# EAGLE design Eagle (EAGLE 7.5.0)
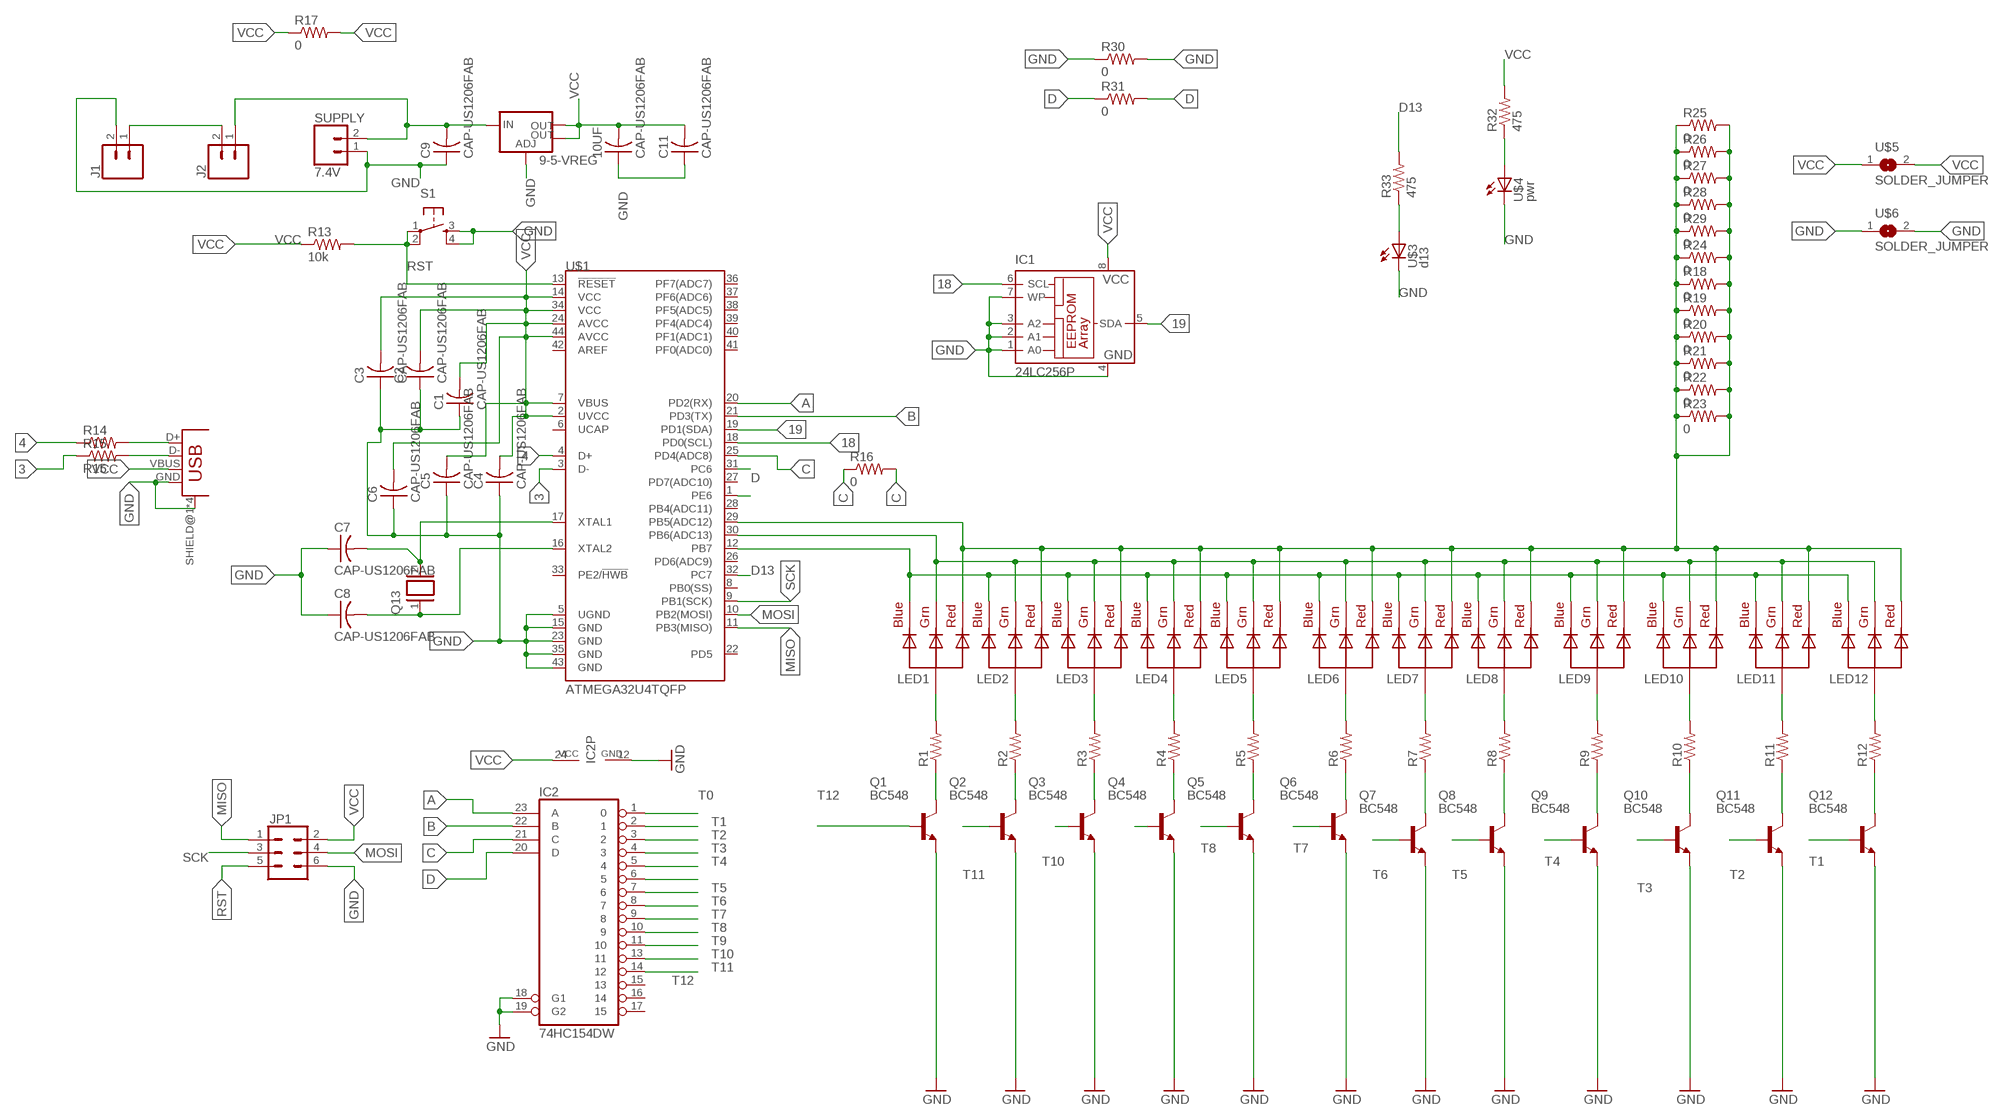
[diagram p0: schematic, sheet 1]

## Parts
9-5-VREG  V_REG_LM1117SOT223  [SOT223]
10UF  CAP-US1206FAB  [C1206FAB]
C1  CAP-US1206FAB  [C1206FAB]
C2  CAP-US1206FAB  [C1206FAB]
C3  CAP-US1206FAB  [C1206FAB]
C4  CAP-US1206FAB  [C1206FAB]
C5  CAP-US1206FAB  [C1206FAB]
C6  CAP-US1206FAB  [C1206FAB]
C7  CAP-US1206FAB  [C1206FAB]
C8  CAP-US1206FAB  [C1206FAB]
C9  CAP-US1206FAB  [C1206FAB]
C11  CAP-US1206FAB  [C1206FAB]
IC1  24LC256P  [DIL8]
IC2  74HC154DW  [SO24W]
J1  CONN_02  [1X02]
J2  CONN_02  [1X02]
JP1  CONN_03X22X3_SILK_MALE_PTH  [2X3]
LED1  RGBLED_CA-5MM  [LED5MMRGB]
LED2  RGBLED_CA-5MM  [LED5MMRGB]
LED3  RGBLED_CA-5MM  [LED5MMRGB]
LED4  RGBLED_CA-5MM  [LED5MMRGB]
LED5  RGBLED_CA-5MM  [LED5MMRGB]
LED6  RGBLED_CA-5MM  [LED5MMRGB]
LED7  RGBLED_CA-5MM  [LED5MMRGB]
LED8  RGBLED_CA-5MM  [LED5MMRGB]
LED9  RGBLED_CA-5MM  [LED5MMRGB]
LED10  RGBLED_CA-5MM  [LED5MMRGB]
LED11  RGBLED_CA-5MM  [LED5MMRGB]
LED12  RGBLED_CA-5MM  [LED5MMRGB]
Q1  BC548  [TO92-EBC]
Q2  BC548  [TO92-EBC]
Q3  BC548  [TO92-EBC]
Q4  BC548  [TO92-EBC]
Q5  BC548  [TO92-EBC]
Q6  BC548  [TO92-EBC]
Q7  BC548  [TO92-EBC]
Q8  BC548  [TO92-EBC]
Q9  BC548  [TO92-EBC]
Q10  BC548  [TO92-EBC]
Q11  BC548  [TO92-EBC]
Q12  BC548  [TO92-EBC]
Q13  XTAL  [Q]
R1  R-US_0207/10  [0207/10]
R2  R-US_0207/10  [0207/10]
R3  R-US_0207/10  [0207/10]
R4  R-US_0207/10  [0207/10]
R5  R-US_0207/10  [0207/10]
R6  R-US_0207/10  [0207/10]
R7  R-US_0207/10  [0207/10]
R8  R-US_0207/10  [0207/10]
R9  R-US_0207/10  [0207/10]
R10  R-US_0207/10  [0207/10]
R11  R-US_0207/10  [0207/10]
R12  R-US_0207/10  [0207/10]
R13  10k  RES-US1206FAB  [R1206FAB]
R14  RES-US1206FAB  [R1206FAB]
R15  R15  RES-US1206FAB  [R1206FAB]
R16  0  RES-US1206FAB  [R1206FAB]
R17  0  RES-US1206FAB  [R1206FAB]
R18  0  RES-US1206FAB  [R1206FAB]
R19  0  RES-US1206FAB  [R1206FAB]
R20  0  RES-US1206FAB  [R1206FAB]
R21  0  RES-US1206FAB  [R1206FAB]
R22  0  RES-US1206FAB  [R1206FAB]
R23  0  RES-US1206FAB  [R1206FAB]
R24  0  RES-US1206FAB  [R1206FAB]
R25  0  RES-US1206FAB  [R1206FAB]
R26  0  RES-US1206FAB  [R1206FAB]
R27  0  RES-US1206FAB  [R1206FAB]
R28  0  RES-US1206FAB  [R1206FAB]
R29  0  RES-US1206FAB  [R1206FAB]
R30  0  RES-US1206FAB  [R1206FAB]
R31  0  RES-US1206FAB  [R1206FAB]
R32  475  RES-US1206FAB  [R1206FAB]
R33  475  RES-US1206FAB  [R1206FAB]
S1  6MM_SWITCH6MM_SWITCH  [6MM_SWITCH]
SUPPLY  7.4V  CONN_02  [1X02]
U$1  ATMEGA32U4TQFP  [SPARKFUN-DIGITALIC_TQFP44]
U$2  USB_MINIB  [USB_MINIB]
U$3  d13  LEDFAB1206  [LED1206FAB]
U$4  pwr  LEDFAB1206  [LED1206FAB]
U$5  SOLDER_JUMPER  [SJFAB]
U$6  SOLDER_JUMPER  [SJFAB]

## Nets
3: R15.1 U$1.3(D-)
4: R14.1 U$1.4(D+)
18: IC1.6(SCL) U$1.18(PD0(SCL))
19: IC1.5(SDA) U$1.19(PD1(SDA))
A: IC2.23(A) U$1.20(PD2(RX))
B: IC2.22(B) U$1.21(PD3(TX))
C: IC2.21(C) R16.1 R16.2 U$1.25(PD4(ADC8))
D: IC2.20(D) R31.1 R31.2 U$1.1(PE6)
D13: R33.2 U$1.32(PC7)
GND: 9-5-VREG.1(ADJ) 10UF.1 C1.1 C2.1 C3.1 C4.1 C5.1 C6.1 C7.1 C8.1 C9.1 C11.1 IC1.1(A0) IC1.2(A1) IC1.3(A2) IC1.4(GND) IC1.7(WP) IC2.12(GND) IC2.18(G1) IC2.19(G2) J1.2 JP1.6 Q1.E Q2.E Q3.E Q4.E Q5.E Q6.E Q7.E Q8.E Q9.E Q10.E Q11.E Q12.E R30.1 R30.2 S1.3(S) S1.4(S1) SUPPLY.1 U$1.5(UGND) U$1.15(GND) U$1.23(GND) U$1.35(GND) U$1.43(GND) U$2.GND U$2.SHIELD@1(SHIELD) U$2.SHIELD@2(SHIELD) U$2.SHIELD@3(SHIELD) U$2.SHIELD@4(SHIELD) U$3.2(C) U$4.2(C) U$6.1 U$6.2
MISO: JP1.1 U$1.11(PB3(MISO))
MOSI: JP1.4 U$1.10(PB2(MOSI))
N$1: J1.1 J2.2
N$2: R32.1 U$4.1(A)
N$3: U$1.31(PC6)
N$4: 9-5-VREG.3(IN) C9.2 J2.1 SUPPLY.2
N$5: R33.1 U$3.1(A)
N$6: LED1.1(RED) LED2.1(RED) LED3.1(RED) LED4.1(RED) LED5.1(RED) LED6.1(RED) LED7.1(RED) LED8.1(RED) LED9.1(RED) LED10.1(RED) LED11.1(RED) LED12.1(RED) R18.1 R18.2 R19.1 R19.2 R20.1 R20.2 R21.1 R21.2 R22.1 R22.2 R23.1 R23.2 R24.1 R24.2 R25.1 R25.2 R26.1 R26.2 R27.1 R27.2 R28.1 R28.2 R29.1 R29.2 U$1.29(PB5(ADC12))
N$12: C7.2 Q13.2 U$1.17(XTAL1)
N$13: C8.2 Q13.1 U$1.16(XTAL2)
N$14: R14.2 U$2.D+
N$15: R15.2 U$2.D-
N$16: Q1.C R1.1
N$17: Q2.C R2.1
N$18: Q3.C R3.1
N$19: Q4.C R4.1
N$20: Q5.C R5.1
N$21: Q6.C R6.1
N$22: Q7.C R7.1
N$23: Q8.C R8.1
N$24: Q9.C R9.1
N$25: Q10.C R10.1
N$26: Q11.C R11.1
N$27: Q12.C R12.1
N$29: LED1.3(GREEN) LED2.3(GREEN) LED3.3(GREEN) LED4.3(GREEN) LED5.3(GREEN) LED6.3(GREEN) LED7.3(GREEN) LED8.3(GREEN) LED9.3(GREEN) LED10.3(GREEN) LED11.3(GREEN) LED12.3(GREEN) U$1.30(PB6(ADC13))
N$31: LED1.2(VCC) R1.2
N$32: LED2.2(VCC) R2.2
N$33: LED3.2(VCC) R3.2
N$34: LED4.2(VCC) R4.2
N$35: LED5.2(VCC) R5.2
N$36: LED6.2(VCC) R6.2
N$37: LED7.2(VCC) R7.2
N$38: LED8.2(VCC) R8.2
N$39: LED9.2(VCC) R9.2
N$40: LED10.2(VCC) R10.2
N$41: LED11.2(VCC) R11.2
N$42: LED12.2(VCC) R12.2
N$46: LED1.4(BLUE) LED2.4(BLUE) LED3.4(BLUE) LED4.4(BLUE) LED5.4(BLUE) LED6.4(BLUE) LED7.4(BLUE) LED8.4(BLUE) LED9.4(BLUE) LED10.4(BLUE) LED11.4(BLUE) LED12.4(BLUE) U$1.12(PB7)
RST: JP1.5 R13.2 S1.1(P) S1.2(P1) U$1.13(!RESET)
SCK: JP1.3 U$1.9(PB1(SCK))
T0: IC2.1
T1: IC2.2 Q12.B
T2: IC2.3 Q11.B
T3: IC2.4 Q10.B
T4: IC2.5 Q9.B
T5: IC2.6 Q8.B
T6: IC2.7 Q7.B
T7: IC2.8 Q6.B
T8: IC2.9 Q5.B
T9: IC2.10 Q4.B
T10: IC2.11 Q3.B
T11: IC2.13 Q2.B
T12: IC2.14 Q1.B
VCC: 9-5-VREG.2(OUT) 9-5-VREG.4(OUT) 10UF.2 C1.2 C2.2 C3.2 C4.2 C5.2 C6.2 C11.2 IC1.8(VCC) IC2.24(VCC) JP1.2 R13.1 R17.1 R17.2 R32.2 U$1.2(UVCC) U$1.7(VBUS) U$1.14(VCC) U$1.24(AVCC) U$1.34(VCC) U$1.44(AVCC) U$2.VBUS U$5.1 U$5.2
Unconnected: IC2.15 IC2.16 IC2.17 U$1.6(UCAP) U$1.8(PB0(SS)) U$1.22(PD5) U$1.26(PD6(ADC9)) U$1.27(PD7(ADC10)) U$1.28(PB4(ADC11)) U$1.33(PE2/!HWB) U$1.36(PF7(ADC7)) U$1.37(PF6(ADC6)) U$1.38(PF5(ADC5)) U$1.39(PF4(ADC4)) U$1.40(PF1(ADC1)) U$1.41(PF0(ADC0)) U$1.42(AREF)

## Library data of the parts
9-5-VREG = fab:V_REG_LM1117: Voltage Regulator LM1117 Standard adjustable voltage regulator but in SMD form. Spark Fun Electronics SKU : COM-00595; PROD_ID: VREG-08170
10UF C1-C9 C11 = fab:CAP-US
IC1 = microchip:24*: Serial EEPROM I2C; MF: MICROCHIP; MPN: 24LC256-E/P; OC_FARNELL: 9757970; OC_NEWARK: 92C7169
IC2 = 74xx-eu:74*154: 4-line to 16-line data SELECTOR/MULTIPLEXER
J1 J2 SUPPLY = SparkFun-Connectors:CONN_02: Multi connection point. Often used as Generic Header-pin footprint for 0.1 inch spaced/style header connections
JP1 = SparkFun-Connectors:CONN_03X2: Multi connection point. Often used as Generic Header-pin footprint for 0.1 inch spaced/style header connections You can populate with any combo of single row headers, but if you'd like an exact match, check these: Header - 2x3 (Male, 0.1") (PRT-12807) Header - 2x3 (Female, 0.1") (PRT-13010) 2x3 Pin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; PROD_ID: CONN-09701
LED1-LED12 = adafruitModified:RGBLED_CA: RGB LED, common-anode 5MM Staggered pins 5mm Piranha package http://www.ladyada.net/library/pcb/eaglelibrary.html
Q1-Q12 = transistor-npn:BC548*: NPN Transistor
Q13 = special:XTAL: CRYSTAL
R1-R12 = adafruit:R-US_: RESISTOR, American symbol
R13-R33 = fab:RES-US: Resistor (US Symbol)
S1 = fab:6MM_SWITCH: OMRON SWITCH
U$1 = SparkFun-Retired:ATMEGA32U4: Atmel 44-pin 8-bit Microcontroller with 32KBytes of ISP Flash and USB Controller ----- Please use the QFN-44-NOPAD_1:1 package for the footprint of all boards using a 32U4. Route traces directly away from the pads as much as possible.; PROD_ID: IC-11161
U$2 = fab:USB_MINIB
U$3 U$4 = fab:LED: LED
U$5 U$6 = fab:SOLDER_JUMPER

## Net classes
0 default: drill 0.406 mm, clearance 0.305 mm

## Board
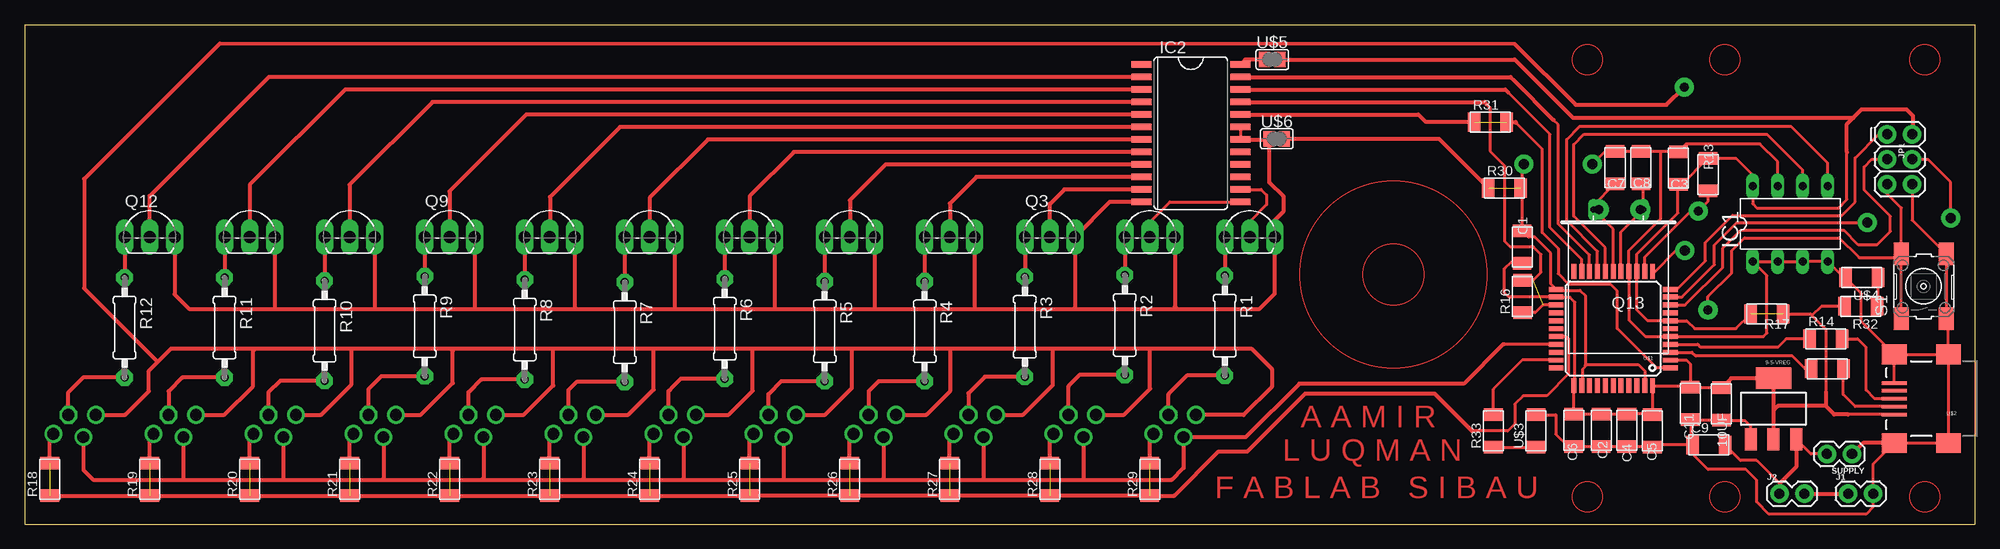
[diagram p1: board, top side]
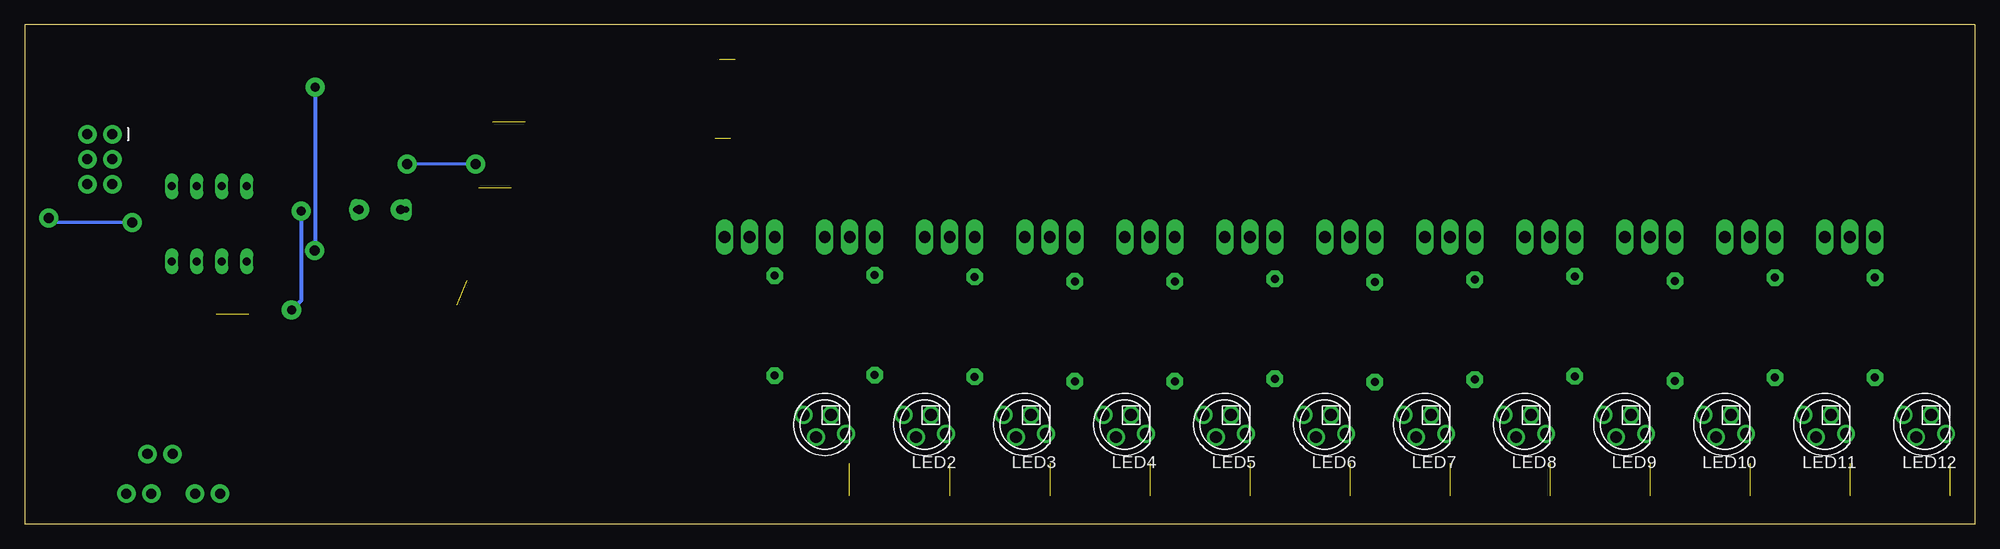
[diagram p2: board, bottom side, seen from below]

Size 198.12 x 50.8 mm. Coordinates in mm from the lower left corner, seen from the top.
Outline: 0,50.8 198.12,50.8 198.12,0 0,0 0,50.8
Copper layers (1*16): Top 0.035mm / dielectric 1.5mm / Bottom 0.035mm
Design rules "default *": minimum track width 10mil, minimum drill 24mil, track to track 12mil, track to pad 12mil, pad to pad 12mil, via to via 12mil, smd to smd 12mil, copper to edge 40mil, drill to drill 8mil, minimum pad ring 10mil, minimum via ring 8mil, stop-mask expansion 4mil, vias tented up to drill 0mil, thermal gap 10mil

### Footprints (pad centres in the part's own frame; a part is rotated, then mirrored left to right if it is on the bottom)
SOT223 = smd 1.219 x 2.235: 1 -2.311,-3.099; 2 0,-3.099; 3 2.311,-3.099 | smd 3.6 x 2.2: 4 0,3.099
C1206FAB = smd 1.27 x 1.905: 1 -1.651,0; 2 1.651,0
DIL8 = drill 0.813 long: 1 -3.81,-3.81; 2 -1.27,-3.81; 3 1.27,-3.81; 4 3.81,-3.81; 5 3.81,3.81; 6 1.27,3.81; 7 -1.27,3.81; 8 -3.81,3.81
SO24W = smd 0.66 x 2.032: 1 -6.985,-5.029; 2 -5.715,-5.029; 3 -4.445,-5.029; 4 -3.175,-5.029; 5 -1.905,-5.029; 6 -0.635,-5.029; 7 0.635,-5.029; 8 1.905,-5.029; 9 3.175,-5.029; 10 4.445,-5.029; 11 5.715,-5.029; 12 6.985,-5.029; 13 6.985,5.029; 14 5.715,5.029; 15 4.445,5.029; 16 3.175,5.029; 17 1.905,5.029; 18 0.635,5.029; 19 -0.635,5.029; 20 -1.905,5.029; 21 -3.175,5.029; 22 -4.445,5.029; 23 -5.715,5.029; 24 -6.985,5.029
1X02 = drill 1.016 pad 1.88: 1 0,0; 2 2.54,0
2X3 = drill 1.016 pad 1.88: 1 0,0; 2 0,2.54; 3 2.54,0; 4 2.54,2.54; 5 5.08,0; 6 5.08,2.54
LED5MMRGB = drill 1.2 pad 1.778: 1 -2.159,0.968; 3 0.889,1.286; 4 2.159,-0.968 | drill 1.2 pad 1.778 octagon: 2 -0.635,-0.968
TO92-EBC = drill 1.2 long: B 0,-1.27; C -2.54,-1.27; E 2.54,-1.27
Q = drill 0.61 long: 1 -2.54,-7.62; 2 2.54,-7.62
0207/10 = drill 0.813 pad 1.676 octagon: 1 -5.08,0; 2 5.08,0
R1206FAB = smd 1.27 x 1.905: 1 -1.651,0; 2 1.651,0
6MM_SWITCH = smd 2.286 x 1.524: 1 -3.302,2.286; 2 3.302,2.286; 3 -3.302,-2.286; 4 3.302,-2.286
SPARKFUN-DIGITALIC_TQFP44 = smd 1.5 x 0.5: 1 -5.8,4; 2 -5.8,3.2; 3 -5.8,2.4; 4 -5.8,1.6; 5 -5.8,0.8; 6 -5.8,0; 7 -5.8,-0.8; 8 -5.8,-1.6; 9 -5.8,-2.4; 10 -5.8,-3.2; 11 -5.8,-4; 23 5.8,-4; 24 5.8,-3.2; 25 5.8,-2.4; 26 5.8,-1.6; 27 5.8,-0.8; 28 5.8,0; 29 5.8,0.8; 30 5.8,1.6; 31 5.8,2.4; 32 5.8,3.2; 33 5.8,4 | smd 0.5 x 1.5: 12 -4,-5.8; 13 -3.2,-5.8; 14 -2.4,-5.8; 15 -1.6,-5.8; 16 -0.8,-5.8; 17 0,-5.8; 18 0.8,-5.8; 19 1.6,-5.8; 20 2.4,-5.8; 21 3.2,-5.8; 22 4,-5.8; 34 4,5.8; 35 3.2,5.8; 36 2.4,5.8; 37 1.6,5.8; 38 0.8,5.8; 39 0,5.8; 40 -0.8,5.8; 41 -1.6,5.8; 42 -2.4,5.8; 43 -3.2,5.8; 44 -4,5.8
USB_MINIB = smd 2.5 x 0.35: D+ 3.77,0; D- 3.77,0.8; GND 3.77,-1.6; ID 3.77,-0.8; VBUS 3.77,1.6 | smd 2.5 x 2: SHIELD@1 -1.73,-4.5; SHIELD@2 -1.73,4.5; SHIELD@3 3.77,4.5; SHIELD@4 3.77,-4.5
LED1206FAB = smd 1.27 x 1.905: 1 -1.651,0; 2 1.651,0
SJFAB = smd 1.118 x 1.6: 1 -0.787,0; 2 0.787,0

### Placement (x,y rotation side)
9-5-VREG  177.65,11.76 0 top
10UF  172.38,12.22 90 top
C1  152.13,28.21 270 top
C2  160.16,9.55 90 top
C3  168.01,36.2 270 top
C4  162.76,9.55 90 top
C5  165.36,9.49 90 top
C6  157.37,9.55 90 top
C7  161.57,36.27 270 top
C8  164.2,36.27 270 top
C9  171.08,8.06 0 top
C11  169.19,12.29 90 top
IC1  179.35,30.55 0 top
IC2  118.47,39.76 270 top
J1  185.25,3.12 0 top
J2  178.27,3.12 0 top
JP1  189.22,39.65 270 top
LED1  116.84,10.16 180 bottom
LED2  106.68,10.16 180 bottom
LED3  96.52,10.16 180 bottom
LED4  86.36,10.16 180 bottom
LED5  76.2,10.16 180 bottom
LED6  66.04,10.16 180 bottom
LED7  55.88,10.16 180 bottom
LED8  45.72,10.16 180 bottom
LED9  35.56,10.16 180 bottom
LED10  25.4,10.16 180 bottom
LED11  15.24,10.16 180 bottom
LED12  5.08,10.16 180 bottom
Q1  124.46,30.48 0 top
Q2  114.3,30.48 0 top
Q3  104.14,30.48 0 top
Q4  93.98,30.48 0 top
Q5  83.82,30.48 0 top
Q6  73.66,30.48 0 top
Q7  63.5,30.48 0 top
Q8  53.34,30.48 0 top
Q9  43.18,30.48 0 top
Q10  33.02,30.48 0 top
Q11  22.86,30.48 0 top
Q12  12.7,30.48 0 top
Q13  161.92,24.38 180 top
R1  121.92,20.2 270 top
R2  111.76,20.26 270 top
R3  101.6,20.07 270 top
R4  91.44,19.61 270 top
R5  81.28,19.61 270 top
R6  71.12,19.87 270 top
R7  60.96,19.55 270 top
R8  50.8,19.81 270 top
R9  40.64,20.13 270 top
R10  30.48,19.68 270 top
R11  20.32,20 270 top
R12  10.16,20 270 top
R13  171.01,35.55 270 top
R14  182.97,18.87 0 top
R15  183.1,15.82 0 top
R16  152.16,23.14 90 top
R17  177,21.39 180 top
R18  2.54,4.57 90 top
R19  12.7,4.57 90 top
R20  22.86,4.57 90 top
R21  33.02,4.57 90 top
R22  43.18,4.57 90 top
R23  53.34,4.57 90 top
R24  63.5,4.57 90 top
R25  73.66,4.57 90 top
R26  83.82,4.57 90 top
R27  93.98,4.57 90 top
R28  104.14,4.57 90 top
R29  114.3,4.57 90 top
R30  150.34,34.19 0 top
R31  148.91,40.88 0 top
R32  186.55,22.16 180 top
R33  149.22,9.49 90 top
S1  192.91,24.18 90 top
SUPPLY  185.64,7.15 180 top
U$1  161.38,19.89 180 top
U$2  193.7,12.77 180 top
U$3  153.53,9.49 90 top
U$4  186.62,25.09 180 top
U$5  126.75,47.26 0 top
U$6  127.2,39.2 0 top

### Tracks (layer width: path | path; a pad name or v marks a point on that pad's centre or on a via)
3
  Top 0.305: U$1.3 169.38,17.49 169.78,17.09 179.59,17.09 180.96,15.73 181.37,15.73 R15.1
4
  Top 0.305: U$1.4 169.95,18.29 170.24,18 178.1,18 178.96,18.87 R14.1
18
  Top 0.305: U$1.18 160.57,28.12 157.37,31.33 157.37,38.61 158.41,39.65 177,39.65 180.62,36.02 IC1.6
19
  Top 0.305: U$1.19 159.78,27.75 156.65,30.88 156.65,39.13 157.95,40.43 179.47,40.43 183.16,36.73 IC1.5
A
  Top 0.305: U$1.20 158.97,27.38 155.81,30.55 155.81,40.62 155.32,41.11 | 151.29,45.14 151.06,45.37
  Top 0.406: 155.32,41.11 151.29,45.14 150.96,45.48 IC2.23
B
  Top 0.305: U$1.21 158.18,26.95 154.96,30.16 154.96,39.65 150.7,43.91 150.47,44.13 149.24,44.13
  Top 0.406: IC2.22 150.41,44.2 150.7,43.91
C  (1 unrouted)
  Top 0.305: U$1.25 154.24,22.29 153.47,21.52 152.19,21.52 R16.1 | R16.2 153.23,24.79 154.05,25.61 154.05,27.43 153.27,28.21 150.93,28.21 150.34,28.8 150.34,36.47 148.85,37.96 148.85,42.38 148.53,42.7 148.36,42.87
  Top 0.406: IC2.21 148.29,42.94 148.53,42.7
D  (1 unrouted)
  Top 0.305: 151.51,40.82 154.18,38.16 154.18,29.64 155.81,28.02 155.81,25.48 156.84,24.44 161.07,24.44 161.78,23.73 161.78,19.89 165.78,15.89 U$1.1
  Top 0.406: IC2.20 141.57,41.66 142.35,40.88 R31.1 | R31.2 151.45,40.88 151.51,40.82
D13
  Top 0.305: U$1.32 152.15,16.69 149.22,13.76 R33.2
GND  (via drill 1.02 pad 1.93)  (3 unrouted)
  Top 0.305: C5.1 165.29,7.9 C4.1 C2.1 C6.1 156.81,7.9 155.54,9.16 155.54,11.12 155.52,11.14 U$3.2 | U$2.GND U$2.SHIELD@4 | IC2.19 IC2.18 | IC1.1 IC1.2 IC1.3 IC1.4 184.81,25.09 U$4.2 186.6,23.46 186.6,20.61 U$2.SHIELD@4 | U$2.SHIELD@1 U$2.SHIELD@2 U$2.SHIELD@3 187.79,6.14 J1.2 187.79,1.76 187.07,1.04 177.19,1.04 175.96,2.27 175.96,4.49 174.85,5.59 171.01,5.59 169.59,7.02 169.59,7.9 C9.1 | 165.4,7.8 C5.1 | U$2.SHIELD@4 189.92,16.59 | 166.21,37.92 C8.1 C7.1 160.58,37.92 v159.25,36.59 | 166.21,37.92 167.9,37.92 C3.1 168.78,38.67 176.28,38.67 178.09,36.87 IC1.7 | IC2.12 | 152.13,33.97 C1.1 152.8,29.18 153.4,29.18 155.03,27.56 155.03,24.44 155.56,23.9 | 152.13,33.97 151.91,34.19 | 152.13,33.97 152.13,36.43 v152.29,36.59 | U$2.SHIELD@4 U$2.SHIELD@1 | 194.88,17.14 U$2.SHIELD@1 | S1.4 S1.3 195.43,20.64 U$2.SHIELD@1 | S1.4 194.88,28.07 | 175.89,26.39 IC1.1 | 189.87,17.16 189.87,16.66 U$2.SHIELD@4 | 169.26,10.57 10UF.1 172.42,10.53 174.78,10.53 175.33,9.98 9-5-VREG.1 | 169.26,10.57 C11.1 | IC1.1 177,25.29 177,19.43 176.65,19.09 U$1.5 164.66,19.09 162.97,20.78 U$1.15 162.97,27.84 166.21,31.07 166.21,37.92 | 169.26,10.57 169.26,8.23 C9.1 | C9.1 165.58,8.06 C5.1 | JP1.6 191.75,30.92 S1.4 | U$1.43 164.58,15.6 163.93,16.25 158.6,16.25 158.53,16.18 | 155.5,23.9 155.56,23.9 | 155.56,23.9 U$1.23 | 155.56,23.9 156.08,23.9 156.19,23.79 158.01,23.79 158.53,23.27 158.53,16.18 | 158.53,16.18 158.53,16.05 158.28,15.79 158.28,14.76 158.18,14.65 U$1.35
  Top 0.406: U$2.SHIELD@3 186.76,8.27 SUPPLY.1 | Q12.E 15.24,23.37 16.7,21.91 25.48,21.91 | 25.48,21.91 35.62,21.91 | 35.62,21.91 45.76,21.91 | 45.76,21.91 56.03,21.91 | 56.03,21.91 66.17,21.91 | 66.17,21.91 76.18,21.91 | 76.18,21.91 86.39,21.91 | 86.39,21.91 96.59,21.91 | 96.59,21.91 106.8,21.91 | 106.8,21.91 117.06,21.91 | 117.06,21.91 125.45,21.91 127.01,23.46 Q1.E 127,30.93 127.86,31.79 127.86,33.34 126.42,34.78 U$6.1 126.35,39.12 IC2.18 | Q2.E 116.84,22.13 117.06,21.91 | 106.8,21.91 106.68,22.02 Q3.E 110.23,32.76 IC2.12 | Q4.E 96.52,21.98 96.59,21.91 | Q5.E 86.36,21.93 86.39,21.91 | Q6.E 76.2,21.93 76.18,21.91 | Q7.E 66.04,22.04 66.17,21.91 | Q8.E 55.88,22.05 56.03,21.91 | Q9.E 45.72,21.95 45.76,21.91 | Q10.E 35.56,21.96 35.62,21.91 | Q11.E 25.4,21.98 25.48,21.91 | U$6.2 143.69,39.2 R30.1
  Bottom 0.305: v152.29,36.59 v159.25,36.59
MISO
  Top 0.305: JP1.1 188.37,39.65 185.97,37.24 185.97,32.76 184.6,31.39 173.49,31.39 170.75,28.66 170.75,26.78 167.87,23.89 U$1.11
MOSI  (via drill 1.02 pad 1.93)
  Top 0.305: v195.65,31.14 195.65,34.77 193.31,37.11 JP1.4 | U$1.10 168.37,23.09 171.66,26.39 171.66,28.41 173.94,30.68 v187.2,30.68
  Bottom 0.305: v187.2,30.68 195.19,30.68 v195.65,31.14
N$1
  Top 0.406: J2.2 J1.1
N$2
  Top 0.305: U$4.1 188.27,22.23 R32.1
N$4
  Top 0.305: 178.29,4.16 175.96,6.5 174.29,6.5 C9.2 | SUPPLY.2 181.46,7.15 9-5-VREG.3
  Top 0.406: 9-5-VREG.3 179.96,5.82 178.29,4.16 178.29,3.14 J2.1
N$5
  Top 0.305: R33.1 U$3.1
N$6  (12 unrouted)
  Top 0.305: U$1.29 156.6,19.09 156.84,18.85 156.84,15.28 154.63,13.06 152.23,13.06 151.38,12.22 151.38,10.21 150.67,9.49 147.03,9.49
  Top 0.406: R18.2 2.54,8.81 LED12.1 | R19.2 12.7,8.81 LED11.1 | R20.2 22.86,8.81 LED10.1 | R21.2 33.02,8.81 LED9.1 | R22.2 43.18,8.81 LED8.1 | R23.2 53.34,8.81 LED7.1 | R24.2 63.5,8.81 LED6.1 | R25.2 73.66,8.81 LED5.1 | R26.2 83.82,8.81 LED4.1 | R27.2 93.98,8.81 LED3.1 | R28.2 104.14,8.81 LED2.1 | R29.2 114.3,8.81 LED1.1 | R18.1 R19.1 R20.1 R21.1 R22.1 R23.1 R24.1 R25.1 R26.1 R27.1 R28.1 R29.1 116.8,2.92 121.29,7.41 124.22,7.41 130.06,13.26 143.26,13.26 147.03,9.49
N$7  (via drill 0.91 pad 2.03)
  other vias: 164.12,31.98
N$8  (via drill 0.91 pad 2.03)
  other vias: 159.9,31.98
N$12
  Top 0.305: U$1.17 161.38,30 Q13.2 159.38,32.43 C7.2
N$13
  Top 0.305: U$1.16 162.18,29.71 Q13.1 164.46,34.37 C8.2
N$14
  Top 0.305: U$2.D+ 187.95,12.77 187.07,13.65 187.07,18 186.21,18.87 R14.2
N$15
  Top 0.305: 184.66,15.05 R15.2 184.73,15.12 184.73,13.2 185.95,11.97 U$2.D-
N$16
  Top 0.406: Q1.C R1.1
N$17
  Top 0.406: Q2.C R2.1
N$18
  Top 0.406: Q3.C R3.1
N$19
  Top 0.406: Q4.C R4.1
N$20
  Top 0.406: Q5.C R5.1
N$21
  Top 0.406: Q6.C R6.1
N$22
  Top 0.406: Q7.C R7.1
N$23
  Top 0.406: Q8.C R8.1
N$24
  Top 0.406: Q9.C R9.1
N$25
  Top 0.406: Q10.C R10.1
N$26
  Top 0.406: Q11.C R11.1
N$27
  Top 0.406: Q12.C R12.1
N$29
  Top 0.305: U$1.30 150.31,18.29
  Top 0.406: LED12.3 5.97,5.54 6.96,4.55 16.12,4.55 | 16.12,4.55 26.26,4.55 | 26.26,4.55 36.53,4.55 | 36.53,4.55 46.48,4.55 | 46.48,4.55 56.88,4.55 | 56.88,4.55 66.82,4.55 | 66.82,4.55 77.03,4.55 | 77.03,4.55 87.36,4.55 | 87.36,4.55 97.37,4.55 | 97.37,4.55 107.64,4.55 | 107.64,4.55 116.55,4.55 117.73,5.73 LED1.3 124.05,8.87 129.48,14.3 146.19,14.3 150.18,18.29 150.31,18.29 | LED11.3 16.13,4.56 16.12,4.55 | LED10.3 26.29,4.58 26.26,4.55 | LED9.3 36.45,4.63 36.53,4.55 | LED8.3 46.61,4.68 46.48,4.55 | LED7.3 56.77,4.66 56.88,4.55 | LED6.3 66.93,4.66 66.82,4.55 | LED5.3 77.09,4.61 77.03,4.55 | LED4.3 87.25,4.66 87.36,4.55 | LED3.3 97.41,4.59 97.37,4.55 | LED2.3 107.57,4.62 107.64,4.55
N$31
  Top 0.406: R1.2 118.08,15.12 116.2,13.24 LED1.2
N$32
  Top 0.406: R2.2 107.16,15.18 106.05,14.07 LED2.2
N$33
  Top 0.406: R3.2 97.54,14.99 95.88,13.32 LED3.2
N$34
  Top 0.406: R4.2 86.75,14.53 85.73,13.52 85.73,11.14 LED4.2
N$35
  Top 0.406: R5.2 76.87,14.53 75.56,13.23 LED5.2
N$36
  Top 0.406: R6.2 66.66,14.79 65.84,13.97 65.45,13.59 65.41,13.54 LED6.2
N$37
  Top 0.406: R7.2 56.07,14.47 55.24,13.64 LED7.2
N$38
  Top 0.406: R8.2 46.38,14.73 45.09,13.43 LED8.2
N$39
  Top 0.406: R9.2 36.24,15.05 34.91,13.71 34.91,11.15 LED9.2
N$40
  Top 0.406: R10.2 25.97,14.6 24.77,13.39 LED10.2
N$41
  Top 0.406: R11.2 16.03,14.92 14.62,13.52 14.62,11.15 LED11.2
N$42
  Top 0.406: R12.2 5.95,14.92 4.45,13.41 LED12.2
N$46  (via drill 0.91 pad 1.93, 1.02 pad 1.93)
  Top 0.305: U$1.12 165.29,25.61 165.56,25.61 167.76,27.82 v168.68,27.82
  Top 0.406: v168.61,44.46 166.79,42.64 157.56,42.64 151.38,48.81 19.82,48.88 6.04,35.1 6.04,23.98 13.52,16.51 | LED12.4 10.22,11.13 12.61,13.52 12.61,15.6 13.52,16.51 | 13.52,16.51 14.88,17.88 23.46,17.88 | 23.46,17.88 33.22,17.88 | 33.22,17.88 43.23,17.88 | 43.23,17.88 53.69,17.88 | 53.69,17.88 63.96,17.88 | 63.96,17.88 73.91,17.88 | 73.91,17.88 83.85,17.88 | 83.85,17.88 94.06,17.88 | 94.06,17.88 104.33,17.88 | 104.33,17.88 114.47,17.88 | 114.47,17.88 124.61,17.88 126.69,15.79 126.69,13.97 123.83,11.12 119.01,11.12 LED1.4 | LED11.4 20.29,11.13 23.2,14.04 23.2,17.61 23.46,17.88 | LED10.4 30.11,11.13 33.22,14.23 33.22,17.88 | LED9.4 40.25,11.13 43.48,14.37 43.48,17.61 43.23,17.88 | LED8.4 50.71,11.13 53.69,14.11 53.69,17.88 | LED7.4 61.31,11.13 63.9,13.71 63.9,17.81 63.96,17.88 | LED6.4 71.51,11.13 73.97,13.59 73.97,17.81 73.91,17.88 | LED5.4 81.33,11.13 84.05,13.85 84.05,17.68 83.85,17.88 | LED4.4 91.6,11.13 94.06,13.59 94.06,17.88 | LED3.4 101.41,11.13 104.45,14.17 104.45,17.75 104.33,17.88 | LED2.4 111.68,11.13 114.33,13.78 114.33,17.75 114.47,17.88
  Bottom 0.406: v168.61,44.46 168.61,27.89 v168.68,27.82
RST  (via drill 0.91 pad 1.93)
  Top 0.305: S1.1 S1.2 | S1.2 189.93,27.11 186.35,27.11 184.34,29.12 174.72,29.12 173.42,27.82 173.42,25.55 171.01,23.14 v171.01,21.77 | U$1.13 164.57,27.16 169.26,31.85 | R13.2 171.01,32.83 v170.04,31.85 | S1.2 190.63,27.48 190.65,27.5 190.65,32.17 189.09,33.73 189.09,34.44 JP1.5
  Top 0.406: 169.26,31.85 v170.04,31.85
  Bottom 0.406: v170.04,31.85 170.04,22.75 v171.01,21.77
SCK
  Top 0.305: U$1.9 168.67,22.29 172.51,26.13 172.51,28.08 174.33,29.9 184.79,29.9 186.29,28.41 188.18,28.41 189.54,29.77 189.54,31.33 186.88,33.99 186.88,36.34 187.66,37.12 JP1.3
T1
  Top 0.406: IC2.2 24.8,45.48 12.7,33.37 Q12.B
T2
  Top 0.406: IC2.3 32.57,44.2 22.88,34.52 22.88,29.23 Q11.B
T3
  Top 0.406: IC2.4 41.44,42.94 33.02,34.52 Q10.B
T4
  Top 0.406: IC2.5 50.96,41.66 43.16,33.87 43.16,29.23 Q9.B
T5
  Top 0.406: IC2.6 60.48,40.4 53.37,33.28 53.37,29.23 Q8.B
T6
  Top 0.406: IC2.7 69.42,39.12 63.51,33.22 Q7.B
T7
  Top 0.406: IC2.8 78.16,37.85 73.64,33.34 73.64,29.23 Q6.B
T8
  Top 0.406: IC2.9 87.48,36.59 83.85,32.95 83.85,29.24 Q5.B
T9
  Top 0.406: IC2.10 96.67,35.31 93.99,32.63 Q4.B
T10
  Top 0.406: IC2.11 105.62,34.05 104.14,32.56 Q3.B
T11
  Top 0.305: Q2.B 114.3,30.71 116.35,32.76 123.48,32.76 IC2.13
T12
  Top 0.305: Q1.B 124.46,30.8 126.17,32.5 126.17,33.48 125.59,34.05 IC2.14
VCC  (2 unrouted)
  Top 0.305: 157.37,13.59 C6.2 C2.2 C4.2 165.29,11.21 C5.2 165.38,11.16 U$1.44 169.04,14.09 C11.2 | 157.37,13.59 157.37,14.08 U$1.34 | 167.16,16.7 U$1.2 168.82,16.69 169.19,16.32 C11.2 | U$1.24 150.78,23.09 150.34,23.53 150.34,26 151.06,26.71 151.97,26.71 C1.2 | U$1.24 150.94,23.09 | 182.97,13.46 182.97,19.82 181.58,21.22 | 185.12,37.83 185.12,33.02 184.28,32.17 175.96,32.17 175.54,32.59 IC1.8 175.56,34.38 175.56,35.49 173.85,37.21 R13.1 168.3,34.49 168.03,34.49 C3.2 167.96,34.5 167.96,31.66 163.78,27.47 U$1.14 163.78,21.8 164.88,20.69 U$1.7 168.85,20.69 169.65,19.89 173.85,19.89 R17.2 | U$2.VBUS 185.26,11.17 | C11.2 172.31,13.94 10UF.2 | R17.1 181.41,21.39 181.58,21.22 | R32.2 182.52,22.16 181.58,21.22 | U$1.24 155.59,23.07 156.97,23.07 157.5,22.55 157.5,14.76 157.38,14.63 157.38,13.6 157.37,13.59
  Top 0.406: 185.77,41.34 157.3,41.34 151.38,47.26 U$5.2 | 185.77,41.34 186.62,42.19 191.16,42.19 191.81,41.53 191.81,39.71 JP1.2 | 185.12,37.83 185.12,40.69 185.77,41.34 | 10UF.2 173.36,14.85 9-5-VREG.4 177.71,14.79 177.71,11.63 | 177.71,11.63 177.71,8.72 9-5-VREG.2 | 185.26,11.17 183.83,11.17 182.97,12.03 | 182.97,12.03 178.1,12.03 177.71,11.63 | 182.97,13.46 182.97,12.03 | U$5.1 124,47.26 IC2.24
(copper drawn outside any net)
  shapes: Top circle x8

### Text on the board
Top: A A M I R / L U Q M A N | F A B L A B S I B A U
